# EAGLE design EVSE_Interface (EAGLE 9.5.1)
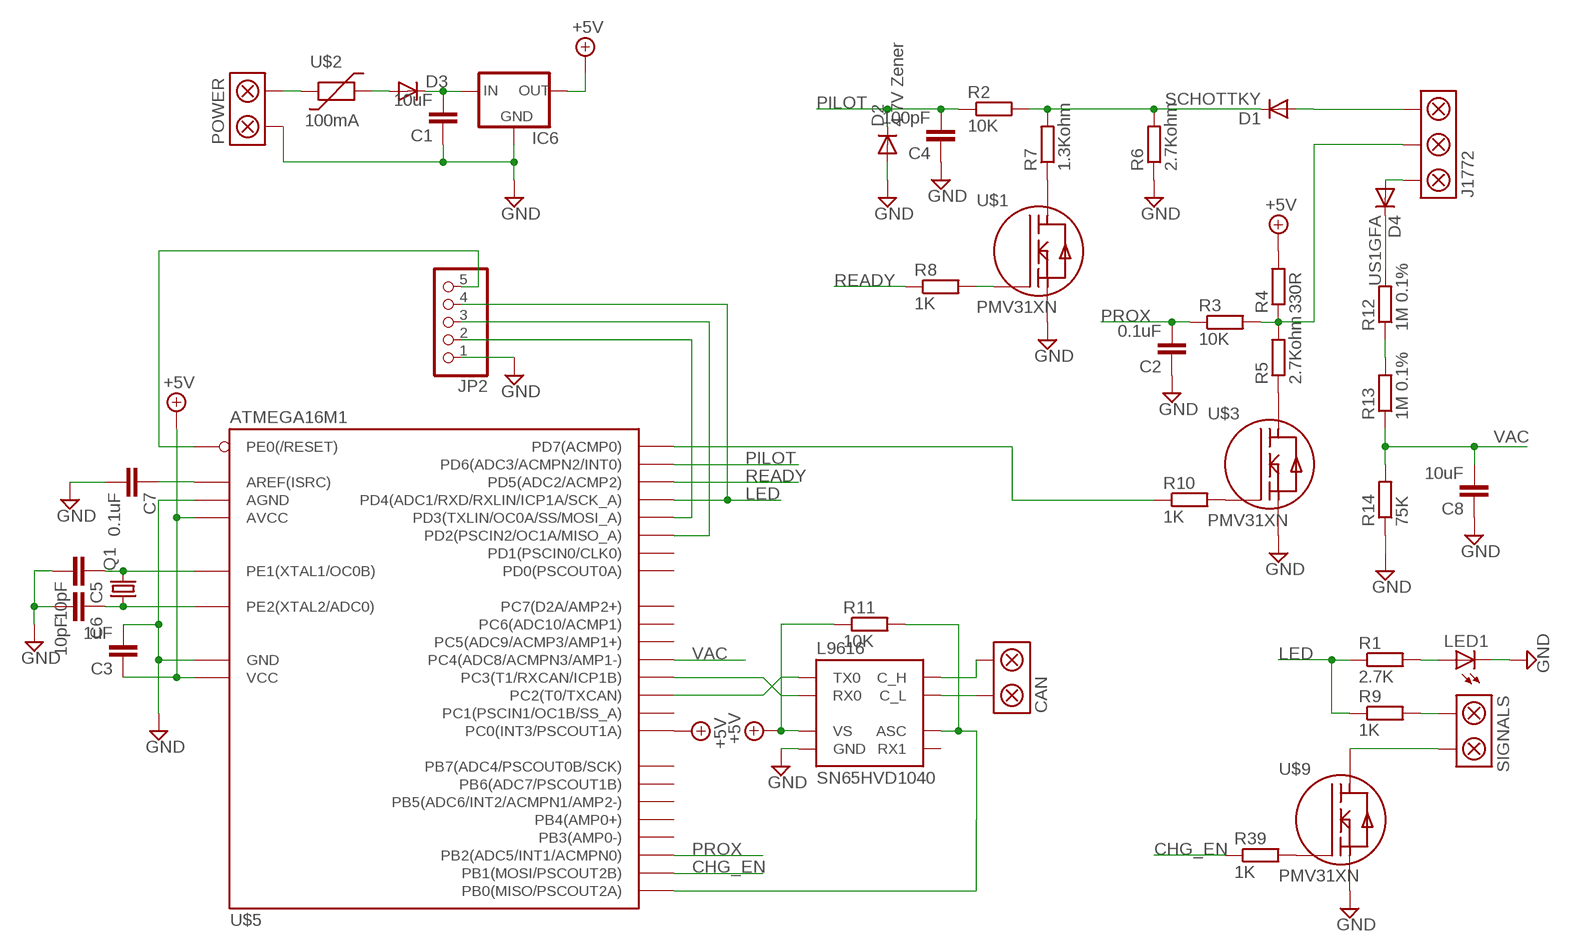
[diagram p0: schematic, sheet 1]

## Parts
C1  10uF  C-EUC1206  [C1206]
C2  0.1uF  C-EUC1206  [C1206]
C3  1uF  C-EUC1206  [C1206]
C4  100pF  C-EUC1206  [C1206]
C5  10pF  C-EUC0805  [C0805]
C6  10pF  C-EUC0805  [C0805]
C7  0.1uF  C-EUC1206  [C1206]
C8  10uF  C-EUC1206  [C1206]
CAN  SCREWTERM_2WAY5MM  [SCREWTERM_5MM_2WAY]
D1  SCHOTTKY  DIODE-SOD123  [SOD123]
D2  4.7V Zener  DIODE-SOD123  [SOD123]
D3  DIODE-SOD123  [SOD123]
D4  US1GFA  DIODE-SOD123  [SOD123]
IC6  78LXXSOT89  [SOT89R]
J1772  SCREWTERM_3WAY5MM  [SCREWTERM_5MM_3WAY]
JP2  PINHD-1X5  [1X05]
LED1  LED3MM  [LED3MM]
POWER  SCREWTERM_2WAY5MM  [SCREWTERM_5MM_2WAY]
Q1  CRYSTALCTS406  [CTS406]
R1  2.7K  R-EU_R1206  [R1206]
R2  10K  R-EU_R1206  [R1206]
R3  10K  R-EU_R1206  [R1206]
R4  330R  R-EU_R1206  [R1206]
R5  2.7Kohm  R-EU_R1206  [R1206]
R6  2.7Kohm  R-EU_R1206  [R1206]
R7  1.3Kohm  R-EU_R1206  [R1206]
R8  1K  R-EU_R1206  [R1206]
R9  1K  R-EU_R1206  [R1206]
R10  1K  R-EU_R1206  [R1206]
R11  10K  R-EU_R1206  [R1206]
R12  1M 0.1%  R-EU_R1206  [R1206]
R13  1M 0.1%  R-EU_R1206  [R1206]
R14  75K  R-EU_R1206  [R1206]
R39  1K  R-EU_R1206  [R1206]
SIGNALS  SCREWTERM_2WAY5MM  [SCREWTERM_5MM_2WAY]
SN65HVD1040  L9616  [SOIC8]
U$1  PMV31XN  [SOT23]
U$2  100mA  1206_POLYSWITCH  [1206]
U$3  PMV31XN  [SOT23]
U$5  ATMEGA16M1  [TQFP32]
U$9  PMV31XN  [SOT23]

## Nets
+5V: C3.1 IC6.2(OUT) R4.2 R11.1 SN65HVD1040.P$3(VS) U$5.4(VCC) U$5.19(AVCC) U$5.30(PC0(INT3/PSCOUT1A))
CHG_EN: R39.1 U$5.9(PB1(MOSI/PSCOUT2B))
GND: C1.1 C2.1 C3.2 C4.1 C5.2 C6.2 C7.2 C8.1 D2.A IC6.4(GND) JP2.1 LED1.K(C) POWER.P$2 R6.1 R14.1 SN65HVD1040.P$2(GND) U$1.P$2(S) U$3.P$2(S) U$5.5(GND) U$5.20(AGND) U$9.P$2(S)
LED: JP2.4 R1.1 R9.1 U$5.12(PD4(ADC1/RXD/RXLIN/ICP1A/SCK_A))
MISO: JP2.3 U$5.1(PD2(PSCIN2/OC1A/MISO_A))
N$1: J1772.P$2 R3.2 R4.1 R5.2
N$2: POWER.P$1 U$2.P$1
N$3: LED1.A R1.2
N$4: D3.A U$2.P$2
N$5: R9.2 SIGNALS.P$2
N$6: R11.2 SN65HVD1040.P$8(ASC) U$5.8(PB0(MISO/PSCOUT2A))
N$7: CAN.P$2 SN65HVD1040.P$6(C_L)
N$8: R7.1 U$1.P$3(D)
N$9: C1.2 D3.C IC6.1(IN)
N$10: CAN.P$1 SN65HVD1040.P$7(C_H)
N$11: SIGNALS.P$1 U$9.P$3(D)
N$12: SN65HVD1040.P$1(TX0) U$5.6(PC2(T0/TXCAN))
N$13: D1.A J1772.P$1
N$14: D1.C R2.2 R6.2 R7.2
N$15: R8.2 U$1.P$1(G)
N$16: C7.1 U$5.21(AREF(ISRC))
N$17: SN65HVD1040.P$4(RX0) U$5.7(PC3(T1/RXCAN/ICP1B))
N$18: R5.1 U$3.P$3(D)
N$19: R10.2 U$3.P$1(G)
N$20: R10.1 U$5.15(PD7(ACMP0))
N$21: C6.1 Q1.1 U$5.11(PE2(XTAL2/ADC0))
N$22: R12.1 R13.2
N$24: D4.C R12.2
N$25: D4.A J1772.P$3
N$34: C5.1 Q1.3 U$5.10(PE1(XTAL1/OC0B))
N$44: JP2.5 U$5.31(PE0(/RESET))
N$57: R39.2 U$9.P$1(G)
OUTPUT: JP2.2 U$5.2(PD3(TXLIN/OC0A/SS/MOSI_A))
PILOT: C4.2 D2.C R2.1 U$5.14(PD6(ADC3/ACMPN2/INT0))
PROX: C2.2 R3.1 U$5.16(PB2(ADC5/INT1/ACMPN0))
READY: R8.1 U$5.13(PD5(ADC2/ACMP2))
VAC: C8.2 R13.1 R14.2 U$5.17(PC4(ADC8/ACMPN3/AMP1-))
Unconnected: SN65HVD1040.P$5(RX1) U$5.3(PC1(PSCIN1/OC1B/SS_A)) U$5.18(PC5(ADC9/ACMP3/AMP1+)) U$5.22(PC6(ADC10/ACMP1)) U$5.23(PB3(AMP0-)) U$5.24(PB4(AMP0+)) U$5.25(PC7(D2A/AMP2+)) U$5.26(PB5(ADC6/INT2/ACMPN1/AMP2-)) U$5.27(PB6(ADC7/PSCOUT1B)) U$5.28(PB7(ADC4/PSCOUT0B/SCK)) U$5.29(PD0(PSCOUT0A)) U$5.32(PD1(PSCIN0/CLK0))

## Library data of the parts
C1-C8 = resistor:C-EU: CAPACITOR, European symbol
CAN POWER SIGNALS = Ians parts:SCREWTERM_2WAY
D1-D4 = diode:DIODE-: DIODE
IC6 = v-reg:78LXX: VOLTAGE REGULATOR
J1772 = Ians parts:SCREWTERM_3WAY
JP2 = pinhead:PINHD-1X5: PIN HEADER
LED1 = led:LED: LED
Q1 = crystal:CRYSTAL: CRYSTAL
R1-R14 R39 = rcl:R-EU_: RESISTOR, European symbol
SN65HVD1040 = Ians parts:L9616
U$1 U$3 U$9 = Ians parts:PMV31XN
U$2 = Ians parts:1206_POLYSWITCH
U$5 = Ians parts:ATMEGA16M1

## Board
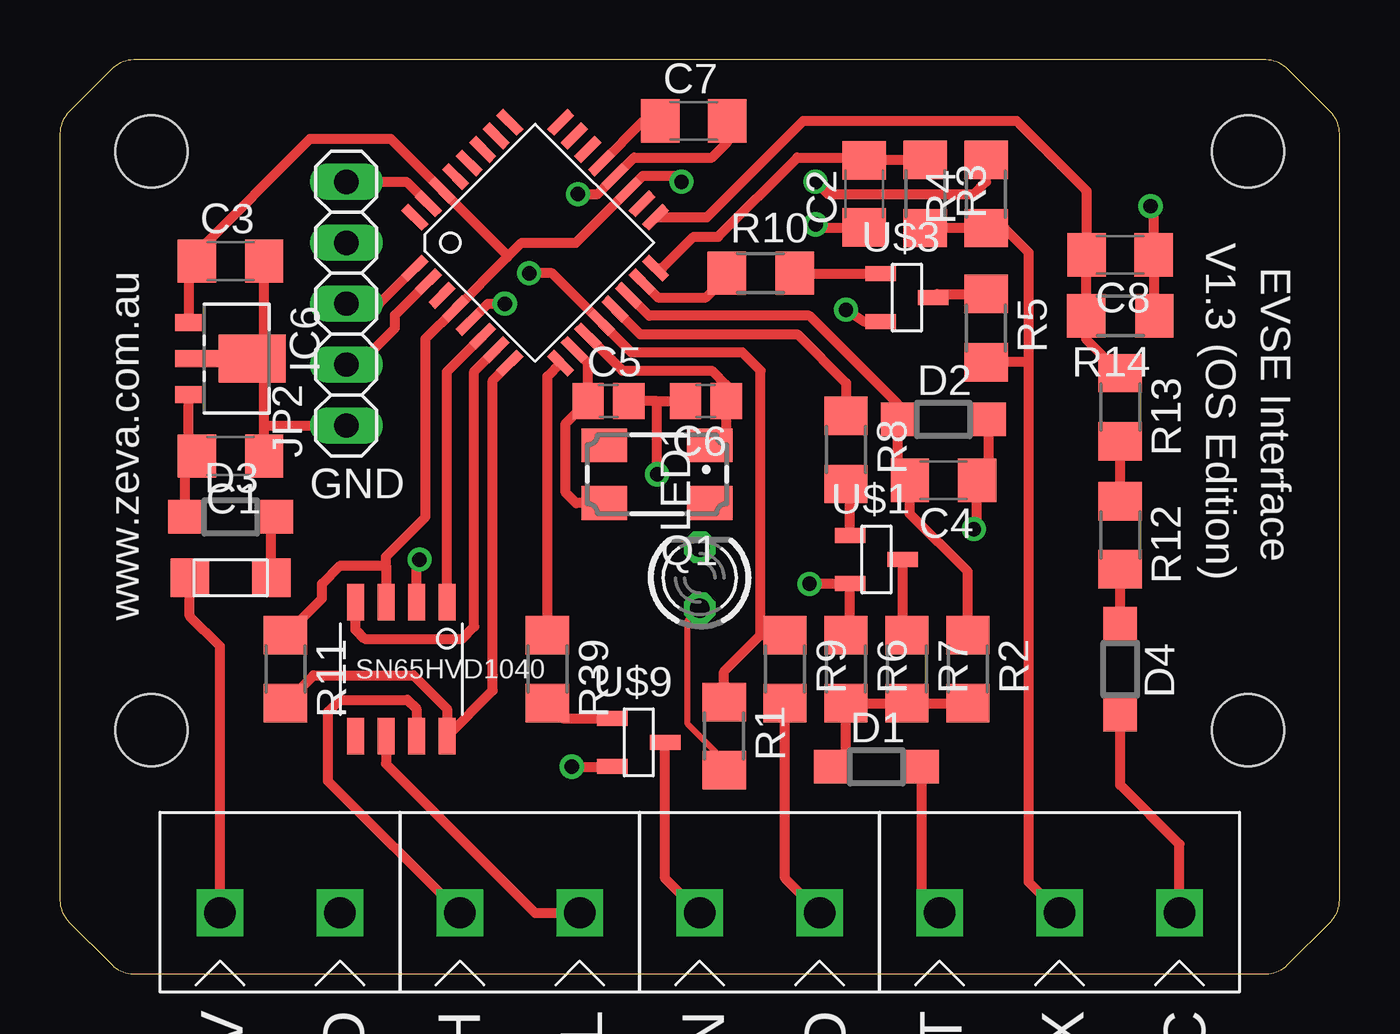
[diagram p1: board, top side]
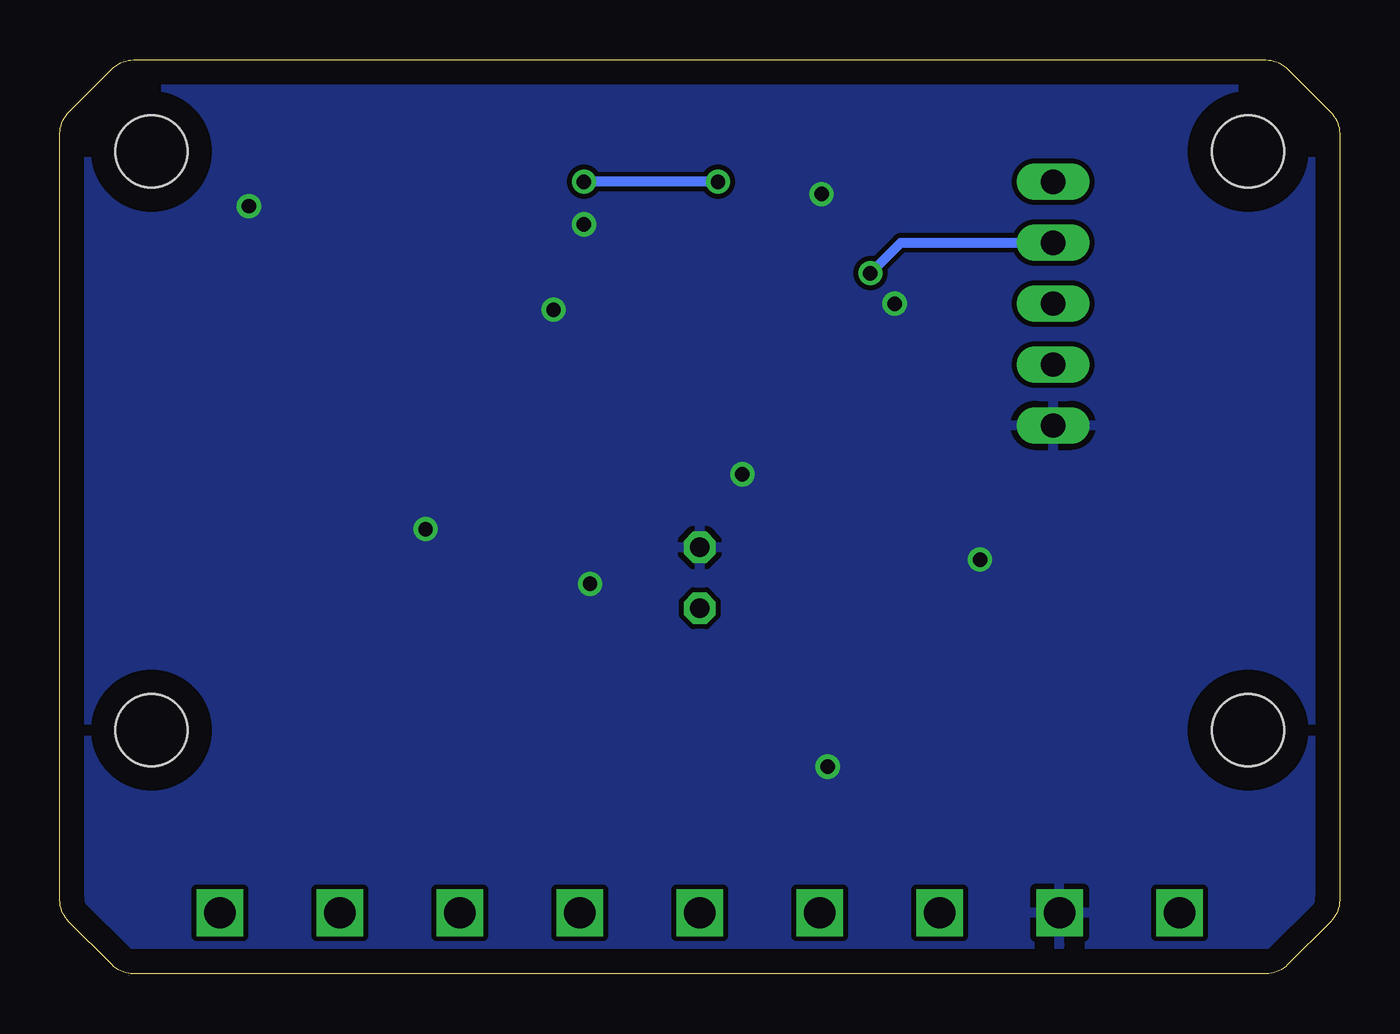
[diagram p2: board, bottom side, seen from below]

Size 53.34 x 38.1 mm. Coordinates in mm from the lower left corner, seen from the top.
Outline: 0.37,35.93 arc45 0,35.03 0,3.07 arc45 0.37,2.17 2.17,0.37 arc45 3.07,0 50.27,0 arc45 51.17,0.37 52.97,2.17 arc45 53.34,3.07 53.34,35.03 arc45 52.97,35.93 51.17,37.73 arc45 50.27,38.1 3.07,38.1 arc45 2.17,37.73 0.37,35.93
Copper layers (1*16): Top 0.035mm / dielectric 1.5mm / Bottom 0.035mm
Design rules "default *": minimum track width 10mil, minimum drill 10mil, track to track 8mil, track to pad 8mil, pad to pad 8mil, via to via 8mil, smd to smd 8mil, copper to edge 40mil, drill to drill 8mil, minimum pad ring 10mil, minimum via ring 8mil, stop-mask expansion 4mil, vias tented up to drill 0mil, thermal gap 10mil
Holes 3 mm at 3.81,10.16 49.53,10.16 3.81,34.29 49.53,34.29

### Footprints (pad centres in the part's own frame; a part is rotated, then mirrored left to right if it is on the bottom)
C1206 = smd 1.6 x 1.8: 1 -1.4,0; 2 1.4,0
C0805 = smd 1.3 x 1.5: 1 -0.85,0; 2 0.85,0
SCREWTERM_5MM_2WAY = drill 1.3 square: P$1 -2.5,0; P$2 2.5,0
SOD123 = smd 1.4 x 1.4: A 1.9,0; C -1.9,0
SOT89R = smd 0.7 x 1.1: 1 1.5,-1.75; 2 -1.5,-1.75 | smd 0.7 x 1.8: 3 0,-1.4 | smd 2 x 2.8: 4 0,0.9
SCREWTERM_5MM_3WAY = drill 1.3 square: P$1 -5,0; P$2 0,0; P$3 5,0
1X05 = drill 1.016 long: 1 -5.08,0; 2 -2.54,0; 3 0,0; 4 2.54,0; 5 5.08,0
LED3MM = drill 0.813 octagon: A -1.27,0; K 1.27,0
CTS406 = smd 1.9 x 1.4: 1 -2.2,-1.2; 2 2.2,-1.2; 3 2.2,1.2; 4 -2.2,1.2
R1206 = smd 1.6 x 1.803: 1 -1.422,0; 2 1.422,0
SOIC8 = smd 1.524 x 0.711: P$1 -2.794,1.905; P$2 -2.794,0.635; P$3 -2.794,-0.635; P$4 -2.794,-1.905; P$5 2.794,-1.905; P$6 2.794,-0.635; P$7 2.794,0.635; P$8 2.794,1.905
SOT23 = smd 1.27 x 0.635: P$1 -1.1,1; P$2 -1.1,-1; P$3 1.1,0
1206 = smd 1.6 x 1.6: P$1 -1.7,0; P$2 1.7,0
TQFP32 = smd 1.2 x 0.4: 1 -4.3,2.8; 2 -4.3,2; 3 -4.3,1.2; 4 -4.3,0.4; 5 -4.3,-0.4; 6 -4.3,-1.2; 7 -4.3,-2; 8 -4.3,-2.8; 17 4.3,-2.8; 18 4.3,-2; 19 4.3,-1.2; 20 4.3,-0.4; 21 4.3,0.4; 22 4.3,1.2; 23 4.3,2; 24 4.3,2.8 | smd 0.4 x 1.2: 9 -2.8,-4.3; 10 -2,-4.3; 11 -1.2,-4.3; 12 -0.4,-4.3; 13 0.4,-4.3; 14 1.2,-4.3; 15 2,-4.3; 16 2.8,-4.3; 25 2.8,4.3; 26 2,4.3; 27 1.2,4.3; 28 0.4,4.3; 29 -0.4,4.3; 30 -1.2,4.3; 31 -2,4.3; 32 -2.8,4.3

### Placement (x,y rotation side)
C1  7.11,21.59 180 top
C2  33.53,32.51 90 top
C3  7.11,29.72 0 top
C4  36.83,20.57 180 top
C5  22.86,23.88 0 top
C6  26.92,23.88 180 top
C7  26.42,35.56 0 top
C8  44.2,29.97 180 top
CAN  19.17,2.54 0 top
D1  34.04,8.64 0 top
D2  36.83,23.11 0 top
D3  7.11,19.05 0 top
D4  44.2,12.7 270 top
IC6  7.11,25.65 270 top
J1772  41.67,2.54 0 top
JP2  11.94,27.94 90 top
LED1  26.67,16.51 90 top
POWER  9.17,2.54 0 top
Q1  24.89,20.83 180 top
R1  27.69,9.91 270 top
R2  37.85,12.7 270 top
R3  36.07,32.51 270 top
R4  38.61,32.51 90 top
R5  38.61,26.92 270 top
R6  32.77,12.7 270 top
R7  35.31,12.7 270 top
R8  32.77,21.84 270 top
R9  30.23,12.7 270 top
R10  29.21,29.21 0 top
R11  9.4,12.7 270 top
R12  44.2,18.29 270 top
R13  44.2,23.62 270 top
R14  44.2,27.43 180 top
R39  20.32,12.7 270 top
SIGNALS  29.17,2.54 0 top
SN65HVD1040  14.22,12.7 270 top
U$1  34.04,17.27 0 top
U$2  7.11,16.51 0 top
U$3  35.31,28.19 0 top
U$5  19.81,30.48 45 top
U$9  24.13,9.65 0 top

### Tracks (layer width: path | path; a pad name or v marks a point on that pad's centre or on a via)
+5V  (via drill 0.6)
  Top 0.406: 13.59,17.02 SN65HVD1040.P$3 | 13.59,17.02 13.59,17.4 15.24,19.05 15.24,26.47 U$5.4 18.64,29.87 | IC6.2 5.36,29.37 C3.1 5.71,30.1 10.41,34.8 13.8,34.8 U$5.30 18.64,29.95 18.64,29.87 | 18.64,29.87 19.25,30.48 20.32,30.48 21.51,30.48 U$5.19 24.3,33.27 25.65,33.27 v25.91,33.02 | 38.61,34.54 R4.2 38.61,33.02 38.1,32.51 32,32.51 v31.5,33.02 | R11.1 10.92,15.65 10.92,16.26 11.68,17.02 13.59,17.02
  Bottom 0.406: v25.91,33.02 v31.5,33.02
CHG_EN
  Top 0.406: U$5.9 20.32,24.91 R39.1
GND  (via drill 0.6)
  Top 0.406: v14.99,17.27 14.86,17.14 SN65HVD1040.P$2 | 24.89,23.88 C5.2 | 24.89,23.88 C6.2 | v24.89,20.83 24.89,23.88 | C1.1 8.51,22.86 | 8.51,22.86 8.51,25.15 IC6.4 8.51,26.15 C3.2 | U$5.5 17.84,27.94 v18.54,27.94 | v21.59,32.51 22.41,32.51 U$5.20 23.93,34.04 27.18,34.04 27.82,34.67 C7.2 | U$9.P$2 23.01,8.64 v21.34,8.64 | 8.51,22.86 JP2.1 | v38.1,18.54 38.23,18.67 C4.1 38.73,21.07 D2.A | R6.1 32.94,14.29 U$1.P$2 32.92,16.26 v31.24,16.26 | C2.1 31.63,31.11 v31.5,31.24 | U$3.P$2 33.51,27.19 v32.77,27.69 | R14.1 45.62,29.95 C8.1 45.6,31.87 v45.47,32
  pour Bottom: -1.27,-1.27 54.61,-1.27 54.36,40.64 -1.27,40.64
LED  (via drill 0.6)
  Top 0.406: 29.21,14.12 R9.1 | v19.56,29.21 20.52,29.21 U$5.12 23.82,25.91 28.45,25.91 29.21,25.15 29.21,14.12 | R1.1 27.69,12.6 29.21,14.12
  Bottom 0.406: v19.56,29.21 18.29,30.48 JP2.4
MISO
  Top 0.406: JP2.3 13.31,27.94 U$5.1
N$1
  Top 0.406: R3.2 R4.1 39.37,31.09 40.39,30.07 40.39,27.69 40.39,27.43 | 40.39,25.5 40.39,24.99 40.39,24.64 40.39,3.82 J1772.P$2 | 40.39,25.5 40.39,26.01 40.39,27.43 | 40.39,25.5 R5.2 | 40.39,25.5 40.39,27.43
N$2
  Top 0.406: U$2.P$1 5.41,14.91 6.67,13.65 POWER.P$1
N$3
  Top 0.254: R1.2 27.69,8.89 26.16,10.41 26.16,14.73 LED1.A
N$4
  Top 0.406: U$2.P$2 8.81,18.85 D3.A
N$5
  Top 0.406: SIGNALS.P$2 30.23,3.98 R9.2
N$6
  Top 0.406: U$5.8 18.03,24.74 18.03,12.45 18.03,11.81 SN65HVD1040.P$8 16.13,11.05 14.73,12.45 10.57,12.45 R11.2
N$7
  Top 0.406: SN65HVD1040.P$6 13.59,8.76 19.81,2.54 CAN.P$2
N$8
  Top 0.406: R7.1 35.14,14.29 U$1.P$3
N$9
  Top 0.406: D3.C 5.21,21.09 C1.2 5.36,21.94 IC6.1
N$10
  Top 0.406: SN65HVD1040.P$7 14.86,11.05 14.48,11.43 11.68,11.43 11.18,10.92 11.18,8.03 CAN.P$1
N$11
  Top 0.406: SIGNALS.P$1 25.23,3.98 U$9.P$3
N$12
  Top 0.406: U$5.6 16.13,25.1 SN65HVD1040.P$1
N$13
  Top 0.406: J1772.P$1 35.94,3.27 D1.A
N$14
  Top 0.406: D1.C 32.77,9.28 R6.2 R7.2 R2.2
N$15
  Top 0.406: R8.2 32.94,20.25 U$1.P$1
N$16
  Top 0.406: U$5.21 24.33,35.56 C7.1
N$17
  Top 0.406: SN65HVD1040.P$4 12.32,14.35 12.7,13.97 16.76,13.97 17.27,14.48 17.27,25.11 U$5.7
N$18
  Top 0.406: R5.1 36.56,28.35 U$3.P$3
N$19
  Top 0.406: U$3.P$1 30.87,29.19 R10.2
N$20
  Top 0.406: U$5.15 24.93,28.19 26.92,28.19 27.79,29.06 R10.1
N$21
  Top 0.406: Q1.1 27.77,22.71 C6.1 27.77,24.55 27.18,25.15 23.45,25.15 U$5.11
N$22
  Top 0.406: R12.1 R13.2
N$24
  Top 0.406: D4.C R12.2
N$25
  Top 0.406: J1772.P$3 46.67,5.4 44.2,7.87 D4.A
N$34
  Top 0.406: Q1.3 21.52,19.63 21.08,20.07 21.08,22.95 C5.1 22.01,25.45 U$5.10
N$44
  Top 0.406: JP2.5 14.44,33.02 U$5.31
N$57
  Top 0.406: R39.2 20.95,10.65 U$9.P$1
OUTPUT
  Top 0.406: U$5.2 13.97,27.47 13.97,26.92 12.45,25.4 JP2.2
PILOT
  Top 0.406: R2.1 37.85,16.76 35.43,19.18 C4.2 34.93,21.07 D2.C 34.93,23.74 31.24,27.43 24.56,27.43 U$5.14
PROX
  Top 0.406: R3.1 33.55,33.93 C2.2 33.4,34.04 30.73,34.04 27.43,30.73 26.42,30.73 25.1,29.42 U$5.16
READY
  Top 0.406: U$5.13 24.19,26.67 30.73,26.67 32.77,24.64 R8.1
VAC
  Top 0.406: R13.1 42.77,26.47 R14.2 42.77,29.95 C8.2 42.8,32.64 39.88,35.56 30.99,35.56 26.97,31.54 U$5.17

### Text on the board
tPlace: V1.3 (OS Edition) | EVSE Interface | GND | www.zeva.com.au | 12V | GND | CANH | CANL | CHG EN | LED | PILOT | PROX | VAC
